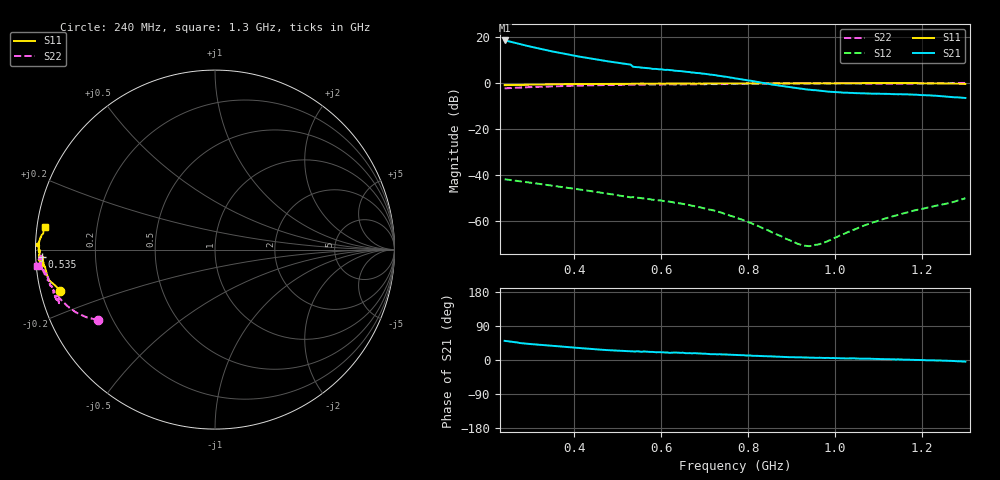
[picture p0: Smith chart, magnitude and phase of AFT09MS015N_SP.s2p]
!Copyright - Freescale Semiconductor, Inc., 2014
! 05/13/2014
! Rev. 0
! AFT09MS015NT1 S-Parameters
! VDD = 12.5 Vdc, IDQ = 400 mA
# Hz  S  MA  R  50.0
!  FREQ  S11M  S11A  S21M  S21A  S12M  S12A  S22M  S22A
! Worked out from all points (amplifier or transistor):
!   213 points, 240 MHz to 1.3 GHz, reference 50 ohm
!   highest |S21| = 18.4 dB at 240 MHz (marker M1)
!   |S21| within 3 dB of that: start of sweep to 307.1 MHz
!   unconditionally stable (mu >= 1): 773.5 MHz to 782 MHz; 812.1 MHz to 823.7 MHz; 826.2 MHz to 1.088 GHz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
!   at 415 MHz: K = 0.14, MSG = 28.8 dB, |S12| = -46.3 dB
!   at 770 MHz: K = 0.88, MSG = 30.1 dB, |S12| = -58.3 dB
!   at 1.3 GHz: K = -0.07, MSG = 21.8 dB, |S12| = -50.1 dB
!   S11 on the Smith chart (normalised r, x): 240 MHz: 0.06, -0.13; 535 MHz: 0.02, -0.02; 1.3 GHz: 0.02, +0.06
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2.4e8  0.8934 -164.9  8.348 50.5  0.008102 -34.4  0.7623 -149.0
2.55e8  0.899 -165.7  7.783 48.2  0.007752 -36.4  0.7761 -150.0
2.8e8  0.9079 -166.9  6.791 44.2  0.00718 -38.9  0.7975 -151.4
2.95e8  0.913 -167.4  6.265 42.6  0.006911 -40.3  0.8085 -152.2
3.1e8  0.918 -167.8  5.829 41.1  0.00661 -41.4  0.8178 -153.0
3.35e8  0.9262 -168.3  5.166 38.9  0.006136 -42.7  0.8327 -154.2
3.55e8  0.9317 -168.8  4.718 37.0  0.0058 -44.2  0.845 -155.2
3.95e8  0.942 -170.1  3.981 33.3  0.005153 -46.6  0.8663 -157.5
4.2e8  0.9458 -171.2  3.617 30.9  0.004763 -48.4  0.879 -158.9
4.7e8  0.9504 -173.4  3.013 26.5  0.004029 -50.9  0.8996 -161.5
5.3e8  0.9554 -174.5  2.498 23.3  0.003272 -51.6  0.9145 -163.8
5.35e8  0.9644 -177.6  2.253 22.7  0.003329 -54.8  0.9189 -161.0
5.95e8  0.9655 -177.0  1.974 20.7  0.002813 -54.2  0.9248 -162.8
6.15e8  0.9691 -176.0  1.929 19.8  0.002681 -54.2  0.9189 -163.8
6.9e8  0.9688 -174.4  1.624 17.3  0.001996 -51.8  0.9378 -167.5
7.7e8  0.9763 -175.2  1.256 13.3  0.001216 -48.3  0.9502 -171.4
8.55e8  0.9731 -177.8  0.9216 9.4  0.0005696 -32.4  0.9716 -173.6
9.15e8  0.9834 -180.0  0.765 7.2  0.0003187 -0.7  0.9728 -174.3
9.5e8  0.9796 179.1  0.6971 6.0  0.0002927 35.3  0.9758 -174.5
1.02e9  0.9856 178.4  0.6145 4.4  0.0005234 78.6  0.9712 -175.8
1.125e9  0.9905 178.7  0.577 2.1  0.001212 89.0  0.9661 -177.7
1.3e9  0.9547 172.6  0.4704 -4.3  0.003136 83.2  0.9987 -174.7
